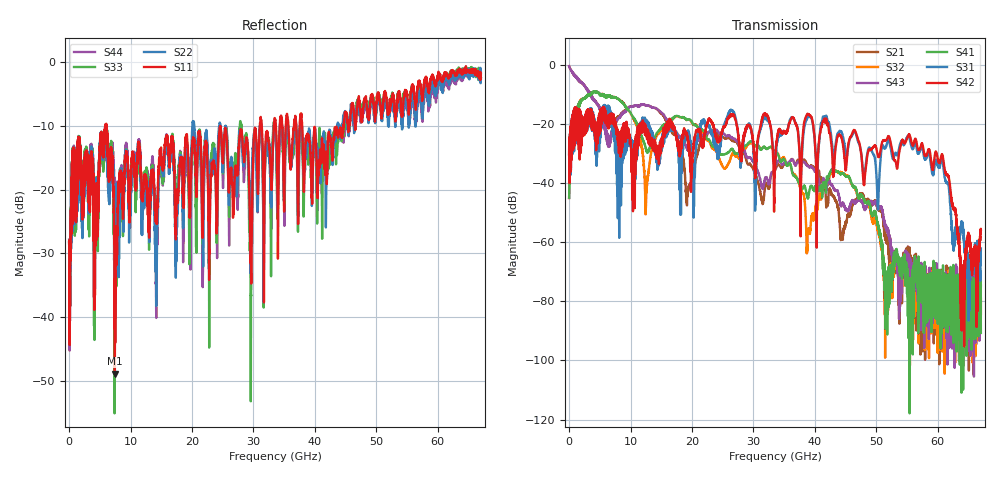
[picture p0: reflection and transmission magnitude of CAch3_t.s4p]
!Agilent Technologies,N5247A,US51170199,A.09.90.13
!Agilent N5247A: A.09.90.13
!Date: Wednesday, October 17, 2018 15:37:25
!Correction: S11(Full 4 Port(1,2,3,4))
!S12(Full 4 Port(1,2,3,4))
!S13(Full 4 Port(1,2,3,4))
!S14(Full 4 Port(1,2,3,4))
!S21(Full 4 Port(1,2,3,4))
!S22(Full 4 Port(1,2,3,4))
!S23(Full 4 Port(1,2,3,4))
!S24(Full 4 Port(1,2,3,4))
!S31(Full 4 Port(1,2,3,4))
!S32(Full 4 Port(1,2,3,4))
!S33(Full 4 Port(1,2,3,4))
!S34(Full 4 Port(1,2,3,4))
!S41(Full 4 Port(1,2,3,4))
!S42(Full 4 Port(1,2,3,4))
!S43(Full 4 Port(1,2,3,4))
!S44(Full 4 Port(1,2,3,4))
!S4P File: Measurements: <S11,S12,S13,S14>,
!<S21,S22,S23,S24>,
!<S31,S32,S33,S34>,
!<S41,S42,S43,S44>:
# Hz S  dB  R 50
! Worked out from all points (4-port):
!   6701 points, 10 MHz to 67 GHz, reference 50 ohm
!   strongest paths, dB at 10 MHz, 16.76 GHz, 33.51 GHz, 50.25 GHz, 67 GHz:
!     S42: -30.2, -20.2, -34.5, -30.7, -55.7
!     S31: -30.3, -21.1, -32.9, -48.7, -62.1
!     S41: -44.9, -18.3, -29.8, -54.5, -90.7
!     S43: -0.4, -21.4, -35.0, -48.1, -74.7
!     S32: -45.1, -18.5, -29.8, -56.2, -84.2
!     S21: -0.4, -22.8, -35.6, -48.8, -79.1
!   lowest |S11| = -48.9 dB at 7.449 GHz (marker M1), VSWR 1.01, Z = 50 - j0.36 ohm
!   |S11| at or under -10 dB: start of sweep to 5.92 GHz; 6.065 GHz to 31.03 GHz (24.97 GHz wide, 135 % of centre); 37.92 GHz to 44.62 GHz (6.702 GHz wide, 16.2 % of centre)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
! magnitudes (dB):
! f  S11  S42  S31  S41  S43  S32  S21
! 10 MHz  -28.3  -30.2  -30.3  -44.9  -0.4  -45.1  -0.4
! 7.449 GHz  -48.9  -19.0  -22.2  -10.9  -20.3  -10.9  -18.7
! 12.55 GHz  -18.3  -23.4  -20.6  -28.5  -13.6  -44.7  -13.6
! 55.14 GHz  -6.3  -24.0  -24.0  -76.3  -65.6  -73.1  -62.7
! 60.79 GHz  -3.0  -30.7  -33.0  -77.4  -71.6  -71.6  -75.5
! 63.99 GHz  -1.2  -72.6  -53.8  -85.3  -73.5  -80.2  -77.1
! 67 GHz  -2.6  -55.7  -62.1  -90.7  -74.7  -84.2  -79.1
